ORGANIZATION_BLOCK "OB Not Loaded Fault"
TITLE =
VERSION : 0.1


VAR_TEMP
  OB85_EV_CLASS : BYTE ;	//16#35 Event class 3
  OB85_FLT_ID : BYTE ;	//16#XX, Fault identification code
  OB85_PRIORITY : BYTE ;	//26 (Priority of 1 is lowest)
  OB85_OB_NUMBR : BYTE ;	//85 (Organization block 85, OB85)
  OB85_RESERVED_1 : BYTE ;	//Reserved for system
  OB85_RESERVED_2 : BYTE ;	//Reserved for system
  OB85_RESERVED_3 : INT ;	//Reserved for system
  OB85_ERR_EV_CLASS : BYTE ;	//Class of event causing error
  OB85_ERR_EV_NUM : BYTE ;	//Number of event causing error
  OB85_OB_PRIOR : BYTE ;	//Priority of OB causing error
  OB85_OB_NUM : BYTE ;	//Number of OB causing error
  OB85_DATE_TIME : DATE_AND_TIME ;	//Date and time OB85 started
END_VAR
BEGIN
END_ORGANIZATION_BLOCK

